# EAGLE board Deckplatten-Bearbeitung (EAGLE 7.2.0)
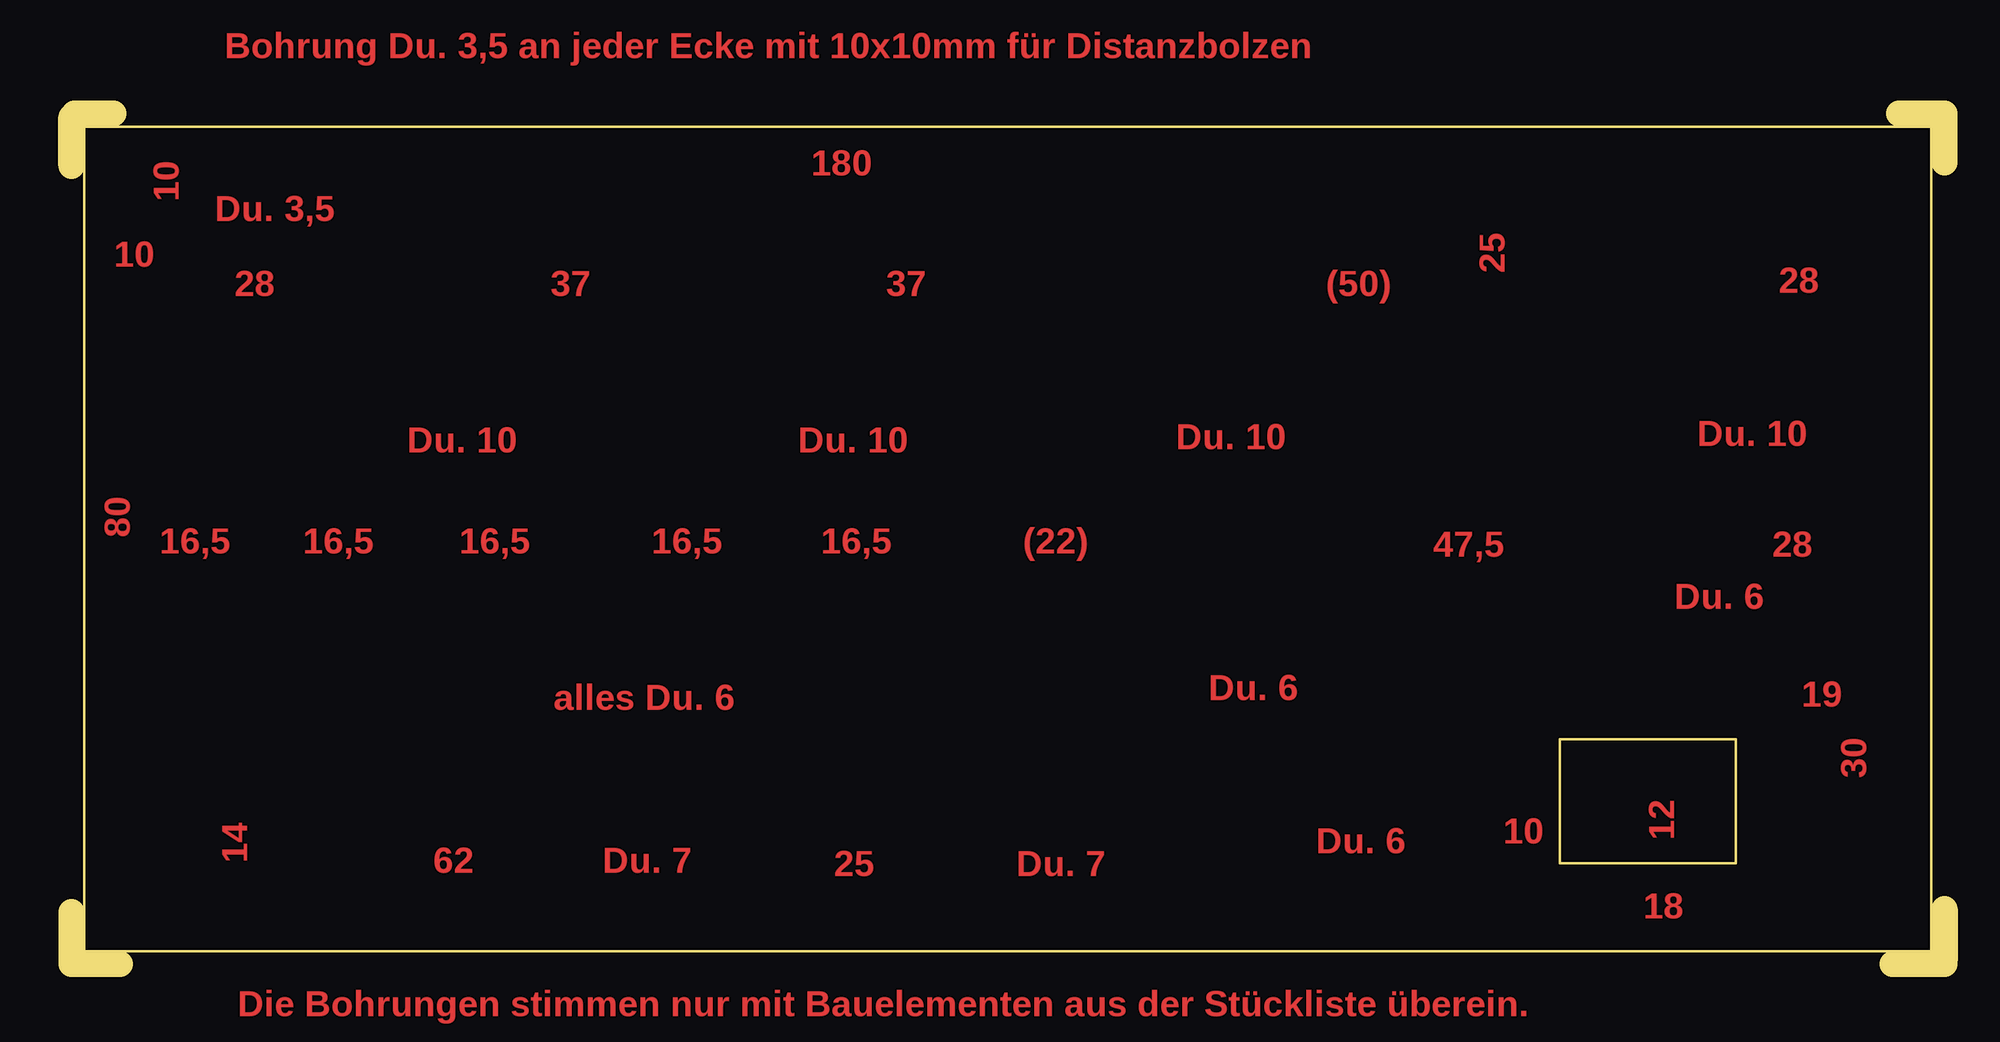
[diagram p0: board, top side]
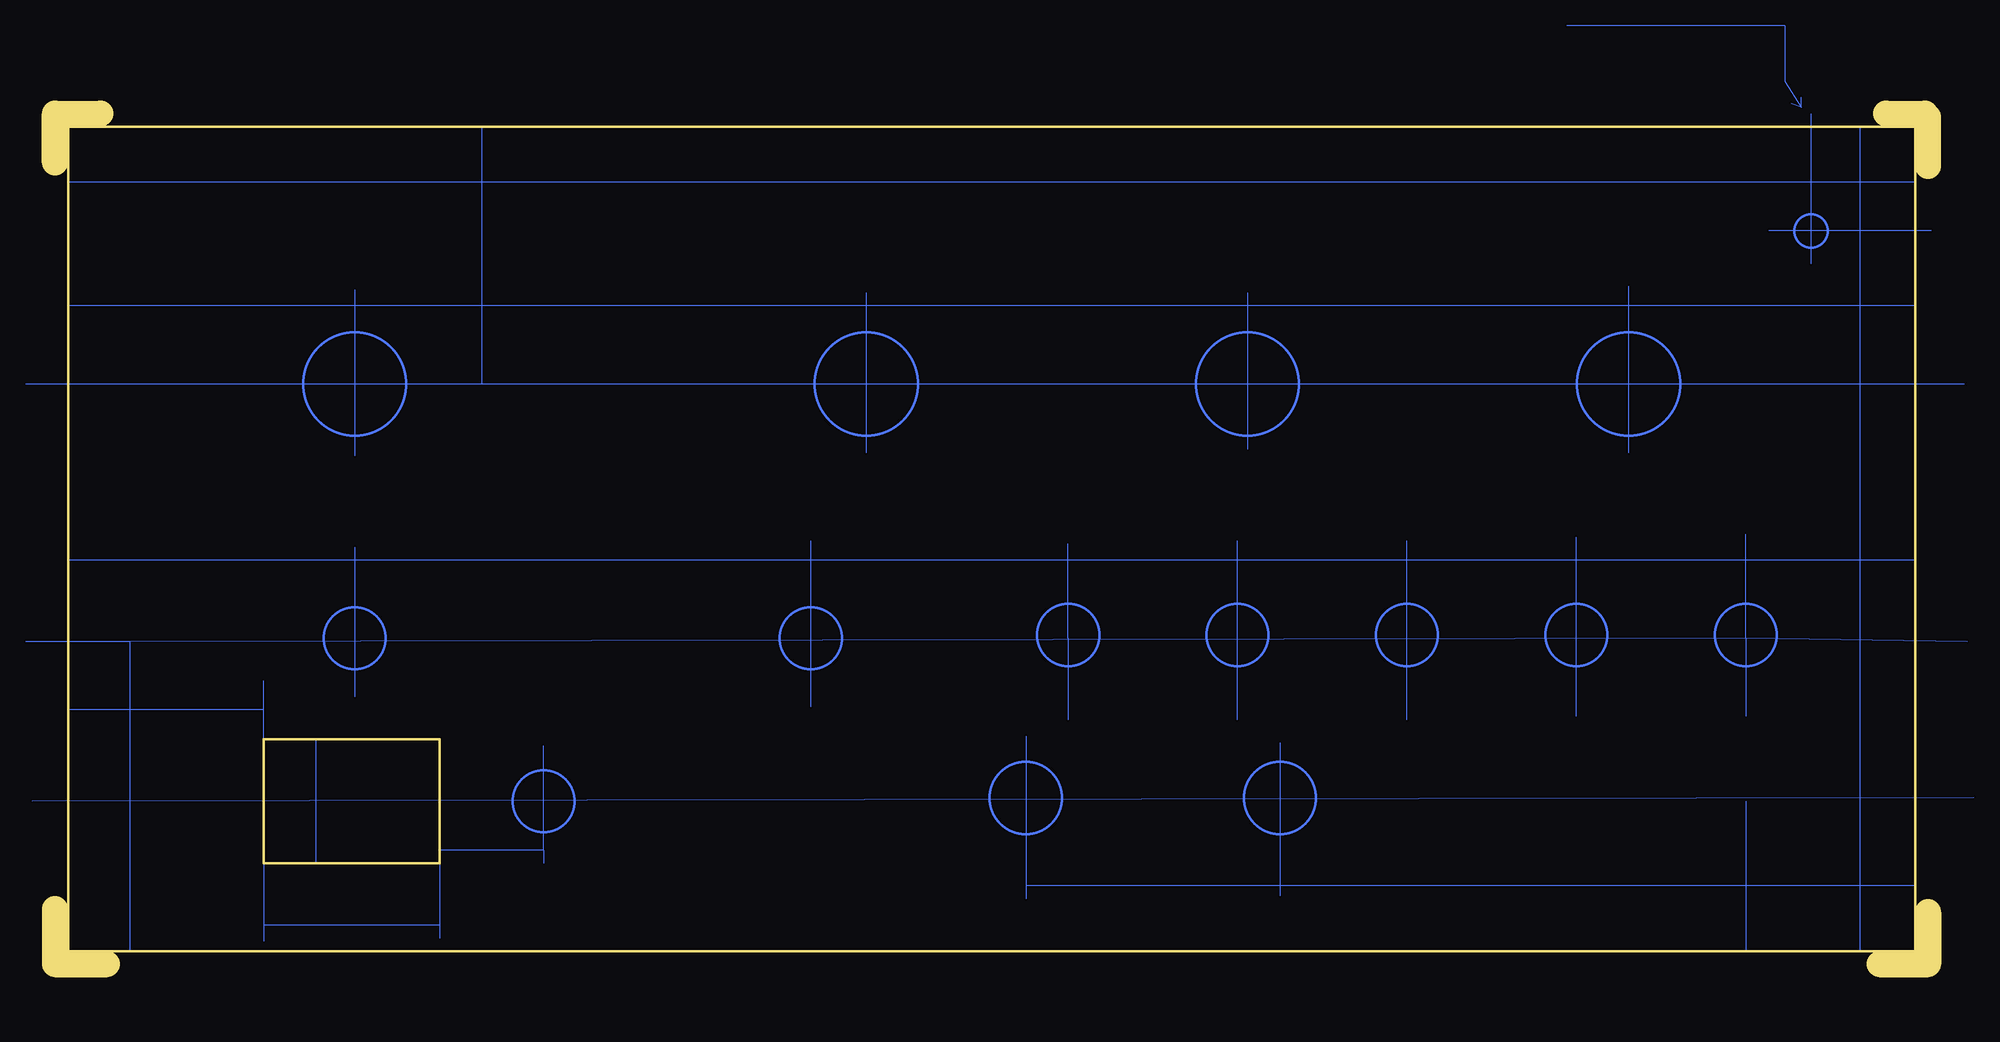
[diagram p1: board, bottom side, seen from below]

Size 182.56 x 82.87 mm. Coordinates in mm from the lower left corner, seen from the top.
Outline: 182.56,5.4 182.56,0.32
Outline: 182.56,0 177.48,0
Outline: 182.56,78.1 182.56,82.87 178.12,82.87
Outline: 0,5.08 0,0 4.76,0
Outline: 4.13,82.87 0.32,82.87
Outline: 0,77.79 0,82.55
Outline: 181.29,1.27 181.29,81.6 1.27,81.6 1.27,1.27 181.29,1.27
Outline: 162.24,21.91 162.24,9.84 145.1,9.84 145.1,21.91 162.24,21.91
Copper layers (1*16): Top 0.035mm / dielectric 1.5mm / Bottom 0.035mm
Design rules "default": minimum track width 10mil, minimum drill 24mil, track to track 8mil, track to pad 8mil, pad to pad 8mil, via to via 8mil, smd to smd 8mil, copper to edge 40mil, drill to drill 8mil, minimum pad ring 10mil, minimum via ring 8mil, stop-mask expansion 4mil, vias tented up to drill 0mil, thermal gap 10mil

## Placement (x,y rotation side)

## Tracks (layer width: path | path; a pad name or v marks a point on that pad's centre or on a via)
S$1
  Bottom 0: -3.49,56.52 140.97,56.52 | 140.97,56.52 185.42,56.52 | 140.97,81.6 140.97,56.52
S$2
  Bottom 0: 29.21,66.04 29.21,49.85
S$3
  Bottom 0: 66.36,65.41 66.36,50.17
S$4
  Bottom 0: 103.5,65.41 103.5,49.85
S$5
  Bottom 0: 153.35,65.72 153.35,49.53
S$6
  Bottom 0: 1.27,64.77 1.27,64.14 181.29,64.14
S$7
  Bottom 0: 1.27,76.2 181.29,76.2
S$8
  Bottom 0: 6.67,81.6 6.67,1.27
S$9
  Bottom 0: -3.81,31.43 17.78,31.75 | 17.78,31.75 175.26,31.43 | 175.26,31.43 185.42,31.43 | 175.26,31.43 175.26,1.27 | 17.78,31.75 17.78,41.91 | 17.78,31.75 17.78,24.13 | 34.29,24.13 34.29,41.59 | 50.8,23.81 50.8,41.28 | 67.31,23.81 67.31,41.28
S$10
  Bottom 0: 153.35,40.64 153.35,26.04
S$11
  Bottom 0: 108.9,41.28 108.9,25.08
S$12
  Bottom 0: 1.27,39.37 181.29,39.37
S$13
  Bottom 0: -4.45,16.19 184.78,15.88
S$14
  Bottom 0: 63.18,21.59 63.18,6.67 | 87.95,22.22 87.95,6.35
S$15
  Bottom 0: 1.27,7.62 87.95,7.62
S$16
  Bottom 0: 17.78,15.88 17.78,1.27
S$17
  Bottom 0: 145.1,10.16 145.1,3.81 | 145.1,3.81 145.1,2.54 | 162.24,9.84 162.24,3.81 | 162.24,3.81 162.24,2.22 | 145.1,3.81 162.24,3.81
S$18
  Bottom 0: 156.84,21.91 157.16,21.91 157.16,9.84
S$19
  Bottom 0: 134.94,11.11 134.94,21.27 | 134.94,11.11 134.94,9.84 | 134.94,11.11 145.1,11.11
S$20
  Bottom 0: 83.82,40.96 83.82,31.75 83.82,23.81
S$21
  Bottom 0: 162.24,21.59 162.24,24.77 | 162.24,24.77 162.24,27.62 | 162.24,24.77 181.29,24.77
S$22
  Bottom 0: 11.43,82.87 11.43,68.26
S$23
  Bottom 0: -0.32,71.44 15.56,71.44
S$24
  Bottom 0: 12.38,83.5 13.97,86.04 13.97,91.44 35.24,91.44 | 12.38,83.5 13.33,83.82 | 12.38,83.5 12.38,84.45
(copper drawn outside any net)
  shapes: Bottom circle x15

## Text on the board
Top: Alles so ungefähr masstabs-getreu ! | Die Abkürzung "Du." heißt Durchmesser | Bohrung Du. 3,5 an jeder Ecke mit 10x10mm für Distanzbolzen | 180 | 10 | Du. 3,5 | 10 | 25 | 28 | 37 | 37 | (50) | 28 | Du. 10 | Du. 10 | Du. 10 | Du. 10 | 80 | 16,5 | 16,5 | 16,5 | 16,5 | 16,5 | (22) | 47,5 | 28 | Du. 6 | Du. 6 | 19 | alles Du. 6 | 30 | 10 | 12 | Du. 6 | 14 | 62 | Du. 7 | 25 | Du. 7 | 18 | Die Bohrungen stimmen nur mit Bauelementen aus der Stückliste überein.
